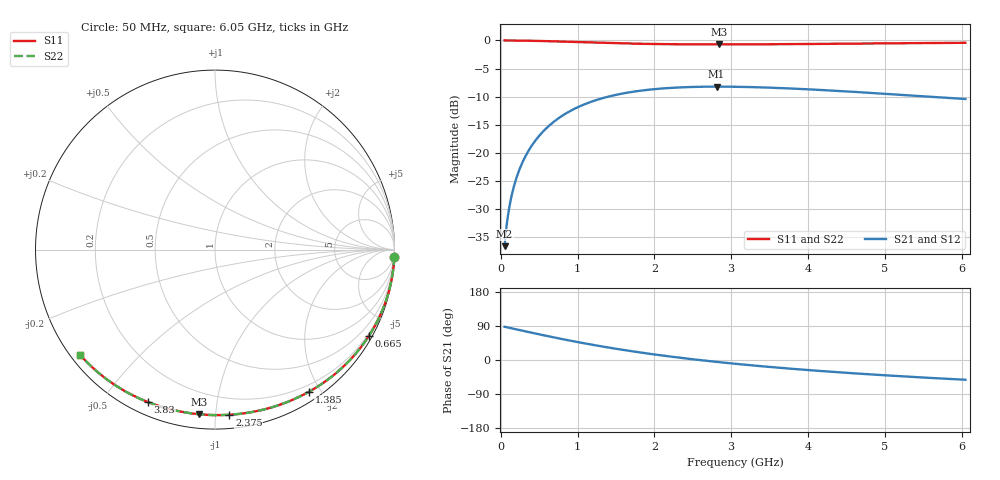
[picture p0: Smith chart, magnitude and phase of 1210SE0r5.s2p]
! AVX Thin Film Operation		Date: August 2001
! Description: Accu-P® Series, Thin Film, SMD, RF Capacitor
! Part Number: 12101J0R5ABT
! 50 MHz  -  6.05 GHz
! Serial Measurements
# mhz S db R 50
!	S11		S21		S12		S22
!	dB	Phase	dB	Phase	dB	Phase	dB	Phase
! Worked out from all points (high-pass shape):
!   401 points, 50 MHz to 6.05 GHz, reference 50 ohm
!   highest |S21| = -8.23 dB at 2.81 GHz (marker M1); lowest = -36.7 dB at 50 MHz (marker M2)
!   |S21| within 3 dB of the highest: 1.117 GHz to end of sweep
!   lowest |S11| = -0.7 dB at 2.84 GHz (marker M3), VSWR 24.52, Z = 3.71 - j45.2 ohm
!   |S11| at or under -10 dB: nowhere
!   |S22| runs from -0.7 to 0.0 dB; largest |S21 - S12| = 0
!   S11 on the Smith chart (normalised r, x): 50 MHz: 0, -51; 665 MHz: 0.13, -3.83; 1.385 GHz: 0.12, -1.85; 2.375 GHz: 0.09, -1.09; 3.83 GHz: 0.05, -0.65; 6.05 GHz: 0.03, -0.34
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50  -0.00 -2.3  -36.66 87.8  -36.66 87.8  -0.00 -2.3
65  -0.00 -2.9  -34.38 87.1  -34.38 87.1  -0.00 -2.9
110  -0.00 -5.0  -29.82 85.0  -29.82 85.0  -0.00 -5.0
140  -0.01 -6.3  -27.74 83.7  -27.74 83.7  -0.01 -6.3
200  -0.01 -9.0  -24.67 81.0  -24.67 81.0  -0.01 -9.0
260  -0.03 -11.7  -22.43 78.3  -22.43 78.3  -0.03 -11.7
335  -0.04 -15.0  -20.29 75.0  -20.29 75.0  -0.04 -15.0
425  -0.07 -19.0  -18.32 71.0  -18.32 71.0  -0.07 -19.0
665  -0.15 -29.2  -14.78 60.7  -14.78 60.7  -0.15 -29.3
845  -0.22 -36.6  -13.04 53.4  -13.04 53.4  -0.22 -36.6
1055  -0.31 -44.7  -11.57 45.2  -11.57 45.2  -0.31 -44.7
1385  -0.45 -56.5  -10.06 33.5  -10.06 33.5  -0.45 -56.5
1700  -0.56 -66.6  -9.19 23.3  -9.19 23.3  -0.56 -66.7
2060  -0.65 -77.0  -8.61 13.0  -8.61 13.0  -0.65 -77.0
2375  -0.69 -85.0  -8.34 4.9  -8.34 4.9  -0.69 -85.1
2810  -0.71 -94.9  -8.23 -5.0  -8.23 -5.0  -0.71 -95.0
2840  -0.71 -95.6  -8.23 -5.6  -8.23 -5.6  -0.71 -95.6
3050  -0.70 -99.9  -8.25 -9.9  -8.25 -9.9  -0.70 -99.9
3830  -0.65 -113.8  -8.60 -23.8  -8.60 -23.8  -0.65 -113.8
4055  -0.62 -117.3  -8.74 -27.4  -8.74 -27.4  -0.62 -117.3
5060  -0.51 -131.0  -9.55 -41.1  -9.55 -41.1  -0.51 -131.0
6050  -0.42 -142.1  -10.43 -52.1  -10.43 -52.1  -0.42 -142.1
